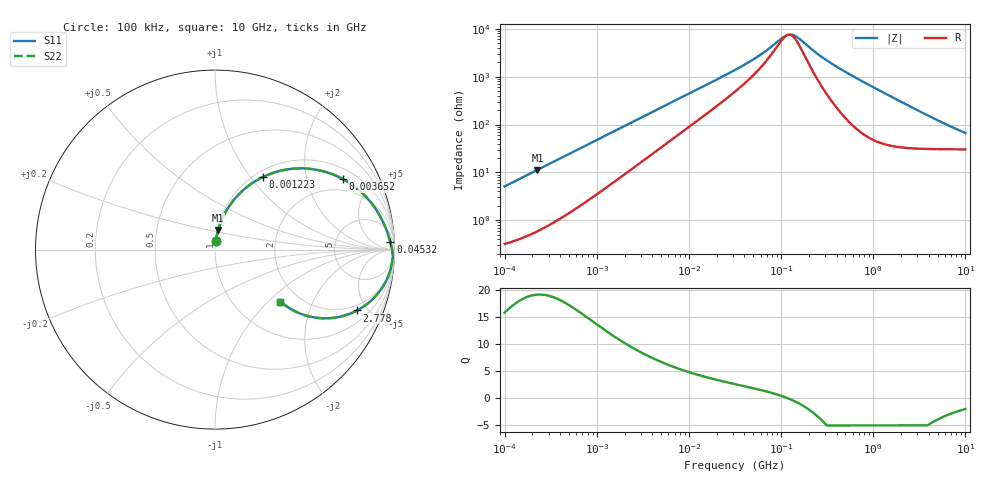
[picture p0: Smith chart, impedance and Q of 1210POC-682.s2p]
# MHz S MA R 50
!Freq  MagS11  AngS11  MagS21  AngS21  MagS12  AngS12  MagS22  AngS22
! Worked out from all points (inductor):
!   801 points, 100 kHz to 10 GHz, reference 50 ohm
!   read as one part in series: L = 8.01 uH near 105.9 kHz
!   highest Q = 19.2 at 227.1 kHz (marker M1), where L = 7.89 uH
!   self-resonance near 119.6 MHz
!   S11 on the Smith chart (normalised r, x): 100 kHz: 1.01, +0.10; 1.223 MHz: 1.09, +1.15; 3.652 MHz: 1.42, +3.31; 45.32 MHz: 19, +37; 2.778 GHz: 1.63, -4.28; 10 GHz: 1.60, -1.19
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0.1  0.05056 83.5  0.9956 -2.9  0.9956 -2.9  0.05056 83.5
0.2271172  0.1114 80.6  0.988 -6.4  0.988 -6.4  0.1114 80.6
0.4278091  0.2021 75.2  0.9682 -11.6  0.9682 -11.6  0.2021 75.2
0.6878599  0.3086 68.4  0.9318 -17.9  0.9318 -17.9  0.3086 68.4
1.223207  0.4848 56.6  0.8372 -28.9  0.8372 -28.9  0.4848 56.6
2.083291  0.6643 42.9  0.6847 -41.4  0.6847 -41.4  0.6643 42.9
3.651741  0.8136 28.9  0.4873 -53.8  0.4873 -53.8  0.8136 28.9
4.663908  0.8582 23.7  0.4058 -58.2  0.4058 -58.2  0.8582 23.7
10  0.9356 12.0  0.2119 -66.4  0.2119 -66.4  0.9356 12.0
31.62278  0.9729 3.8  0.07053 -65.5  0.07053 -65.5  0.9729 3.8
45.31584  0.9781 2.5  0.04783 -61.6  0.04783 -61.6  0.9781 2.5
66.83439  0.9824 1.4  0.02938 -52.5  0.02938 -52.5  0.9824 1.4
104.4119  0.986 0.3  0.01496 -20.6  0.01496 -20.6  0.986 0.3
120.573  0.9869 -0.0  0.01306 1.3  0.01306 1.3  0.9869 -0.0
133.3521  0.9875 -0.2  0.01316 18.7  0.01316 18.7  0.9875 -0.2
147.4857  0.9881 -0.5  0.01449 34.4  0.01449 34.4  0.9881 -0.5
217.5204  0.9896 -1.4  0.02701 66.7  0.02701 66.7  0.9896 -1.4
459.727  0.989 -4.1  0.07161 79.2  0.07161 79.2  0.989 -4.1
1474.857  0.9512 -13.5  0.2342 71.3  0.2342 71.3  0.9512 -13.5
2778.114  0.861 -23.2  0.3983 58.4  0.3983 58.4  0.861 -23.2
5011.872  0.6939 -33.3  0.5675 42.2  0.5675 42.2  0.6939 -33.3
10000  0.4654 -38.5  0.6987 24.5  0.6987 24.5  0.4654 -38.5
